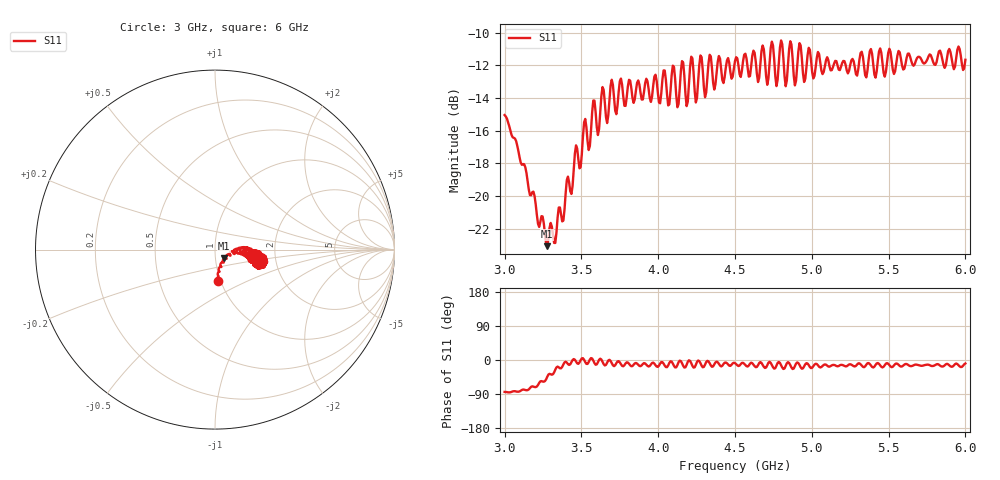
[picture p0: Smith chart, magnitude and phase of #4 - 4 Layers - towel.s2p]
!  02/07/2025  17:16:12
! Ref Plane: 0.000 mm
# MHZ S MA R  50
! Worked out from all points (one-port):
!   401 points, 3 GHz to 6 GHz, reference 50 ohm
!   lowest |S11| = -23.1 dB at 3.277 GHz (marker M1), VSWR 1.15, Z = 55 - j5.43 ohm
!   |S11| at or under -10 dB: start of sweep to end of sweep
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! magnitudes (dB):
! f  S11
! 3 GHz  -15.1
! 3.277 GHz  -23.1
! 3.375 GHz  -21.6
! 3.578 GHz  -14.2
! 3.607 GHz  -16.3
! 3.638 GHz  -13.3
! 3.667 GHz  -15.5
! 3.697 GHz  -12.9
! 3.728 GHz  -15.0
! 3.75 GHz  -13.0
! 4.005 GHz  -14.3
! 4.035 GHz  -12.3
! 4.065 GHz  -14.5
! 4.095 GHz  -12.0
! 4.125 GHz  -14.6
! 4.155 GHz  -11.8
! 4.185 GHz  -14.5
! 4.215 GHz  -11.5
! 4.245 GHz  -14.3
! 4.275 GHz  -11.4
! 4.305 GHz  -14.0
! 4.335 GHz  -11.4
! 4.365 GHz  -13.5
! 4.5 GHz  -11.7
! 4.875 GHz  -11.6
! 5.25 GHz  -12.0
! 5.625 GHz  -11.3
! 6 GHz  -11.7
